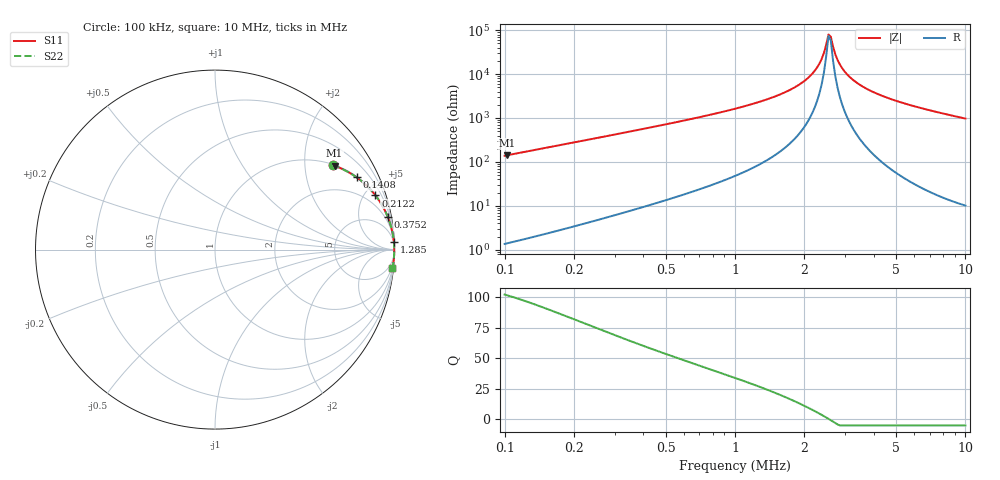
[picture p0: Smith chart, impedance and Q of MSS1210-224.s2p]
# MHz S MA R 50
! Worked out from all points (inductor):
!   203 points, 100 kHz to 10 MHz, reference 50 ohm
!   read as one part in series: L = 220 uH near 102.3 kHz
!   highest Q = 102 at 102.3 kHz (marker M1), where L = 220 uH
!   self-resonance near 2.546 MHz
!   S11 on the Smith chart (normalised r, x): 100 kHz: 1.03, +2.77; 140.8 kHz: 1.04, +3.90; 212.2 kHz: 1.07, +5.90; 375.2 kHz: 1, +11; 1.285 MHz: 3, +47; 10 MHz: 1, -19
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0.1  0.8069 35.6  0.5829 -53.8  0.5829 -53.8  0.8069 35.6
0.102306  0.8132 35.0  0.5741 -54.4  0.5741 -54.4  0.8132 35.0
0.1407715  0.8861 27.0  0.4541 -62.4  0.4541 -62.4  0.8861 27.0
0.2121938  0.9435 18.6  0.3197 -70.6  0.3197 -70.6  0.9435 18.6
0.3751953  0.9797 10.7  0.1851 -78.4  0.1851 -78.4  0.9797 10.7
0.7103709  0.9935 5.4  0.09358 -83.3  0.09358 -83.3  0.9935 5.4
1.285023  0.9975 2.4  0.0422 -85.4  0.0422 -85.4  0.9975 2.4
1.768173  0.9984 1.2  0.02157 -85.1  0.02157 -85.1  0.9984 1.2
2.07411  0.9987 0.7  0.0122 -83.4  0.0122 -83.4  0.9987 0.7
2.272143  0.9988 0.4  0.007025 -79.7  0.007025 -79.7  0.9988 0.4
2.43298  0.9988 0.2  0.003267 -68.7  0.003267 -68.7  0.9988 0.2
2.546482  0.9988 0.0  0.001247 -22.4  0.001247 -22.4  0.9988 0.0
2.605203  0.9989 -0.0  0.0014 35.3  0.0014 35.3  0.9989 -0.0
2.726739  0.9989 -0.2  0.003564 71.5  0.003564 71.5  0.9989 -0.2
2.853945  0.9989 -0.3  0.006064 79.2  0.006064 79.2  0.9989 -0.3
3.055966  0.9989 -0.6  0.009917 83.3  0.009917 83.3  0.9989 -0.6
3.424944  0.9988 -0.9  0.0165 85.5  0.0165 85.5  0.9988 -0.9
4.110185  0.9987 -1.6  0.02752 86.4  0.02752 86.4  0.9987 -1.6
5.162633  0.9982 -2.4  0.04264 86.3  0.04264 86.3  0.9982 -2.4
6.787083  0.9971 -3.7  0.06375 85.5  0.06375 85.5  0.9971 -3.7
8.524974  0.9954 -4.9  0.08484 84.5  0.08484 84.5  0.9954 -4.9
10  0.9937 -5.9  0.1021 83.5  0.1021 83.5  0.9937 -5.9
